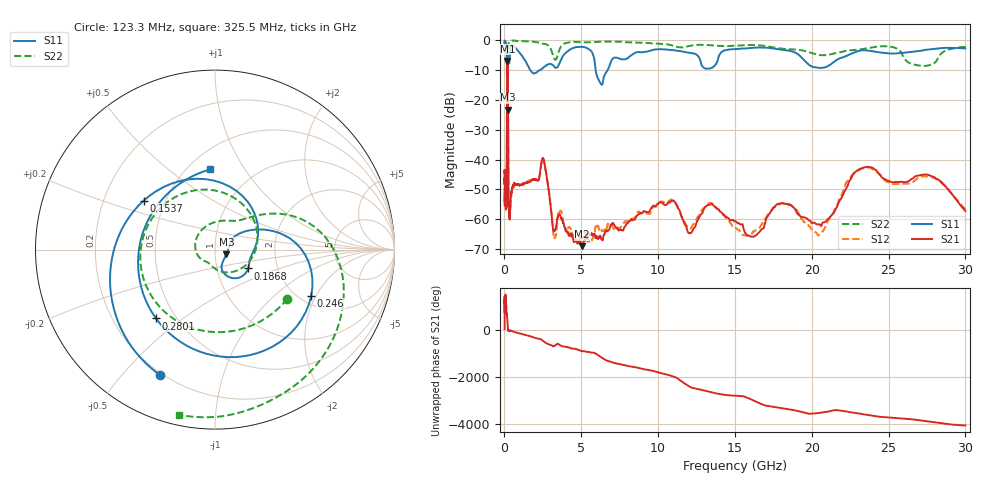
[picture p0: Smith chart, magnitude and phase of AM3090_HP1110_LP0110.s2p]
! Date/Time: Thu, Feb 28, 2019 2:09 PM
! Network Analyzer: Agilent Technologies E8364B Rev: A.07.50.67
! Sweep from 0.010 to 30.000 GHz, 1601 Points, Sweep Type: LOG
! Power Supply: 5.022 V, 0.002 A
# Hz S DB R 50
!freq MagS11 AngS11 MagS21 AngS21 MagS12 AngS12 MagS22 AngS22
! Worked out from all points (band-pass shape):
!   1601 points, 10 MHz to 30 GHz, reference 50 ohm
!   highest |S21| = -7.04 dB at 193.4 MHz (marker M1); lowest = -69.0 dB at 5.052 GHz (marker M2)
!   |S21| within 3 dB of the highest: 172.5 MHz to 219.2 MHz (46.72 MHz wide, 23.9 % of centre)
!   lowest |S11| = -23.3 dB at 212.7 MHz (marker M3), VSWR 1.15, Z = 56.7 - j2.86 ohm
!   |S11| at or under -10 dB: 165.3 MHz to 231.7 MHz (66.47 MHz wide, 33.5 % of centre); 1.669 GHz to 2.36 GHz (691.1 MHz wide, 34.3 % of centre); 5.93 GHz to 6.722 GHz (792.1 MHz wide, 12.5 % of centre)
!   |S22| runs from -21.7 to -0.2 dB; largest |S21 - S12| = 0.012
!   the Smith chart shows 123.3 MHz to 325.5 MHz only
!   S11 on the Smith chart (normalised r, x): 123.3 MHz: 0.19, -0.63; 153.7 MHz: 0.38, +0.27; 186.8 MHz: 1.41, -0.31; 246 MHz: 2.29, -1.83; 280.1 MHz: 0.39, -0.40; 325.5 MHz: 0.64, +0.71
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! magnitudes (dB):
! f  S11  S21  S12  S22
! 10 MHz  -0.3  -44.5  -47.7  -0.6
! 38.04 MHz  -0.3  -52.3  -52.3  -1.2
! 123.3 MHz  -2.3  -53.5  -53.8  -6.2
! 144.7 MHz  -4.5  -49.4  -48.8  -7.5
! 153.7 MHz  -6.3  -33.5  -33.6  -9.0
! 169 MHz  -11.6  -12.2  -12.1  -16.3
! 186.8 MHz  -13.4  -7.2  -7.2  -20.8
! 193.4 MHz  -13.6  -7.0  -7.0  -19.3
! 212.7 MHz  -23.3  -8.4  -8.4  -15.1
! 246 MHz  -4.5  -38.0  -37.9  -2.8
! 280.1 MHz  -5.9  -54.6  -55.0  -1.0
! 325.5 MHz  -7.0  -58.9  -56.5  -0.5
! 550.5 MHz  -2.0  -48.6  -48.9  -0.3
! 2.084 GHz  -10.9  -46.8  -46.9  -0.7
! 2.533 GHz  -9.2  -39.6  -39.8  -1.3
! 3.236 GHz  -8.9  -63.7  -66.4  -6.3
! 5.052 GHz  -2.3  -69.0  -65.8  -0.8
! 6.234 GHz  -14.3  -65.5  -63.5  -0.6
! 7.926 GHz  -6.3  -61.7  -60.7  -0.8
! 20.31 GHz  -9.2  -61.6  -64.5  -4.8
! 23.59 GHz  -3.5  -42.4  -42.7  -2.8
! 30 GHz  -2.8  -57.2  -56.7  -2.3
